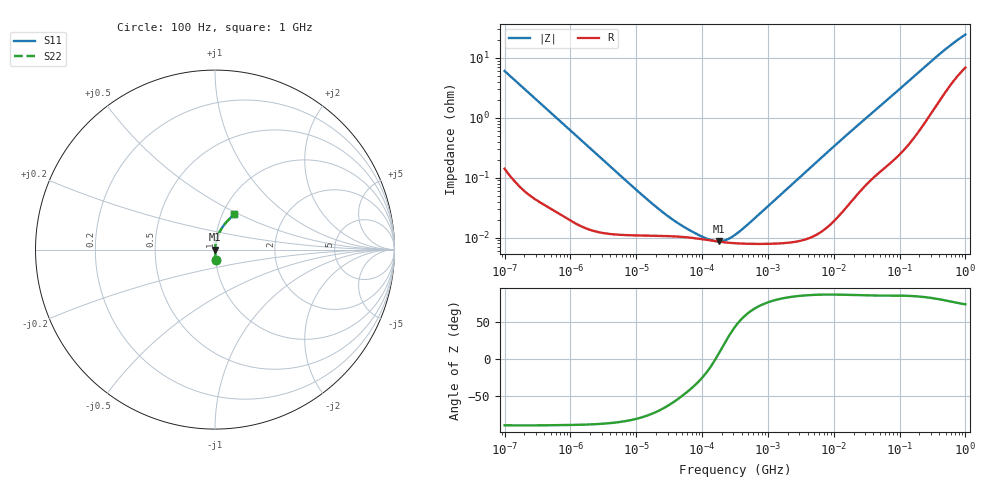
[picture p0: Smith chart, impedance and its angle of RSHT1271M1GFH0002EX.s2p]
! RSHT1271M1GFH0002EX  S-PARAMETER MODEL  (General Type)
! Model Generated by ELNA Corporation (http://www.ty-top.com)
! Version 1.0
! ELNA Control No.201201
! Copyright (c) 2020 ELNA CO.,LTD. All Rights Reserved.
! Products Name : CONDUCTIVE POLYMER HYBRID ALUMINUM ELECTROLYTIC CAPACITORS
! Characteristics :
!  Capacitance  :  270uF  ,  Rated voltage  :  35V
!  Operating Temp. Range  :  -55 to +105 degC  ,  Endurance  :  10000hr at 105 degC
!  Dimension D  :  10mm  ,  Dimension L  :  10mm
! Frequency Range : 100Hz - 1GHz
! External Node Assignments :
!  1  o---| |---o  2
# MHz S RI R 50
!Freq[MHz].  S11 Real  S11 Imag  S21 Real  S21 Imag  S12 Real  S12 Imag  S22 Real  S22 Imag
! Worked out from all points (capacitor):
!   401 points, 100 Hz to 1 GHz, reference 50 ohm
!   read as one part in series: C = 264 uF near 108 Hz
!   lowest |Z| = 8.65 mohm at 179.9 kHz (marker M1)
!   series resonance near 159.5 kHz, so ESL is about 3.8 nH
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0.0001  0.00502 -0.0599  0.995 0.0599  0.995 0.0599  0.00502 -0.0599
0.000113  0.00402 -0.0532  0.996 0.0532  0.996 0.0532  0.00402 -0.0532
0.000309  0.000802 -0.0196  0.9992 0.0196  0.9992 0.0196  0.000802 -0.0196
0.001488  0.00017 -0.00414  0.9998 0.00414  0.9998 0.00414  0.00017 -0.00414
0.009495  0.000109 -0.000651  0.9999 0.000651  0.9999 0.000651  0.000109 -0.000651
0.022131  0.000107 -0.000278  0.9999 0.000278  0.9999 0.000278  0.000107 -0.000278
0.031805  0.000106 -0.000192  0.9999 0.000192  0.9999 0.000192  0.000106 -0.000192
0.045709  0.000104 -0.000131  0.9999 0.000131  0.9999 0.000131  0.000104 -0.000131
0.098288  9.44e-05 -4.55e-05  0.9999 4.55e-05  0.9999 4.55e-05  9.44e-05 -4.55e-05
0.115478  9.19e-05 -3.04e-05  0.9999 3.04e-05  0.9999 3.04e-05  9.19e-05 -3.04e-05
0.179887  8.57e-05 1.19e-05  0.9999 -1.19e-05  0.9999 -1.19e-05  8.57e-05 1.19e-05
0.258523  8.21e-05 5.12e-05  0.9999 -5.12e-05  0.9999 -5.12e-05  8.21e-05 5.12e-05
0.280221  8.15e-05 6.09e-05  0.9999 -6.09e-05  0.9999 -6.09e-05  8.15e-05 6.09e-05
0.316228  8.07e-05 7.63e-05  0.9999 -7.63e-05  0.9999 -7.63e-05  8.07e-05 7.63e-05
0.555904  7.88e-05 0.000168  0.9999 -0.000168  0.9999 -0.000168  7.88e-05 0.000168
4.704354  0.000105 0.00156  0.9999 -0.00156  0.9999 -0.00156  0.000105 0.00156
17.08048  0.000392 0.00557  0.9996 -0.00557  0.9996 -0.00557  0.000392 0.00557
69.9842  0.00214 0.0212  0.9979 -0.0212  0.9979 -0.0212  0.00214 0.0212
176.8072  0.00772 0.0515  0.9923 -0.0515  0.9923 -0.0515  0.00772 0.0515
395.8221  0.0298 0.1062  0.9702 -0.1062  0.9702 -0.1062  0.0298 0.1062
668.3439  0.066 0.156  0.934 -0.156  0.934 -0.156  0.066 0.156
1000  0.1075 0.1966  0.8925 -0.1966  0.8925 -0.1966  0.1075 0.1966
